FUNCTION "Gest Consensi" : VOID
TITLE =GESTIONE CONSENSI
AUTHOR : MassimoZ
VERSION : 0.1

BEGIN
NETWORK
TITLE ======== Consensi Prima Zona =======

NETWORK
TITLE =Cons Salita Testa Corto Circuito 1
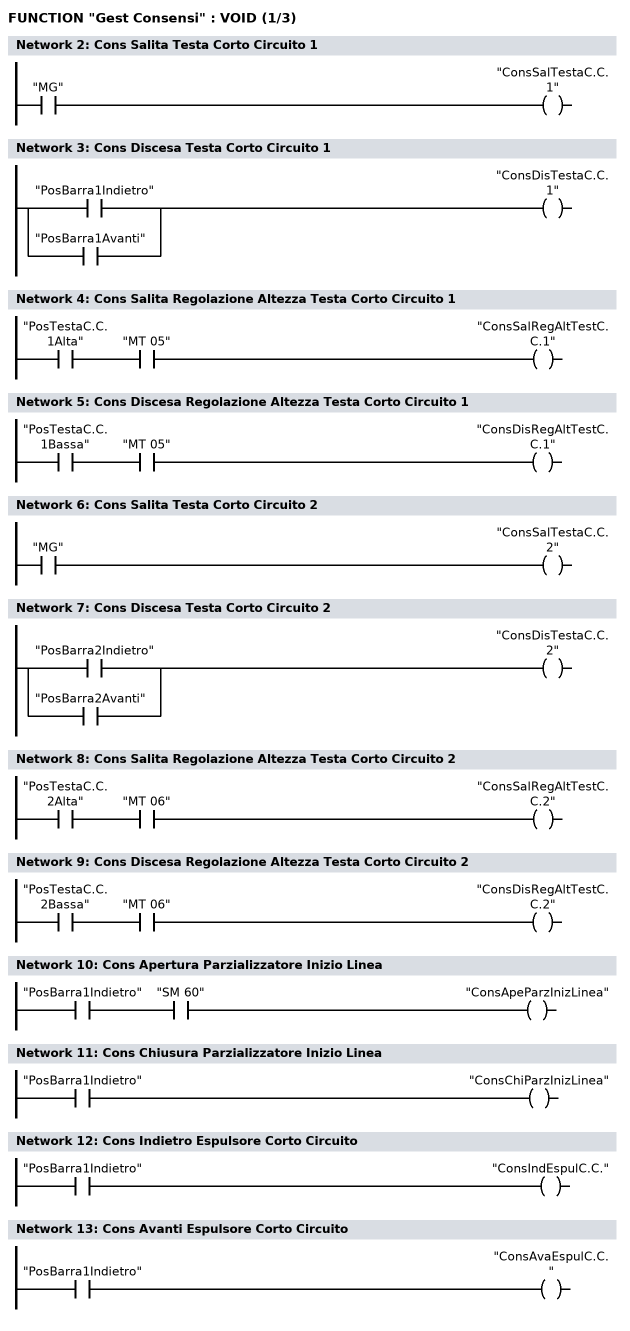
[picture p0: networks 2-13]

      U     "MG";
      =     "ConsSalTestaC.C.1";
NETWORK
TITLE =Cons Discesa Testa Corto Circuito 1

      O     "PosBarra1Indietro";
      O     "PosBarra1Avanti";
      =     "ConsDisTestaC.C.1";
NETWORK
TITLE =Cons Salita Regolazione Altezza Testa Corto Circuito 1

      U     "PosTestaC.C.1Alta";
      U     "MT 05";
      =     "ConsSalRegAltTestC.C.1";
NETWORK
TITLE =Cons Discesa Regolazione Altezza Testa Corto Circuito 1

      U     "PosTestaC.C.1Bassa";
      U     "MT 05";
      =     "ConsDisRegAltTestC.C.1";
NETWORK
TITLE =Cons Salita Testa Corto Circuito 2

      U     "MG";
      =     "ConsSalTestaC.C.2";
NETWORK
TITLE =Cons Discesa Testa Corto Circuito 2

      O     "PosBarra2Indietro";
      O     "PosBarra2Avanti";
      =     "ConsDisTestaC.C.2";
NETWORK
TITLE =Cons Salita Regolazione Altezza Testa Corto Circuito 2

      U     "PosTestaC.C.2Alta";
      U     "MT 06";
      =     "ConsSalRegAltTestC.C.2";
NETWORK
TITLE =Cons Discesa Regolazione Altezza Testa Corto Circuito 2

      U     "PosTestaC.C.2Bassa";
      U     "MT 06";
      =     "ConsDisRegAltTestC.C.2";
NETWORK
TITLE =Cons Apertura Parzializzatore Inizio Linea

      U     "PosBarra1Indietro";
      U     "SM 60";
      =     "ConsApeParzInizLinea";
NETWORK
TITLE =Cons Chiusura Parzializzatore Inizio Linea

      U     "PosBarra1Indietro";
      =     "ConsChiParzInizLinea";
NETWORK
TITLE =Cons Indietro Espulsore Corto Circuito

      U     "PosBarra1Indietro";
      =     "ConsIndEspulC.C.";
NETWORK
TITLE =Cons Avanti Espulsore Corto Circuito

      U     "PosBarra1Indietro";
      =     "ConsAvaEspulC.C.";
NETWORK
TITLE =Cons Indietro Barra 1
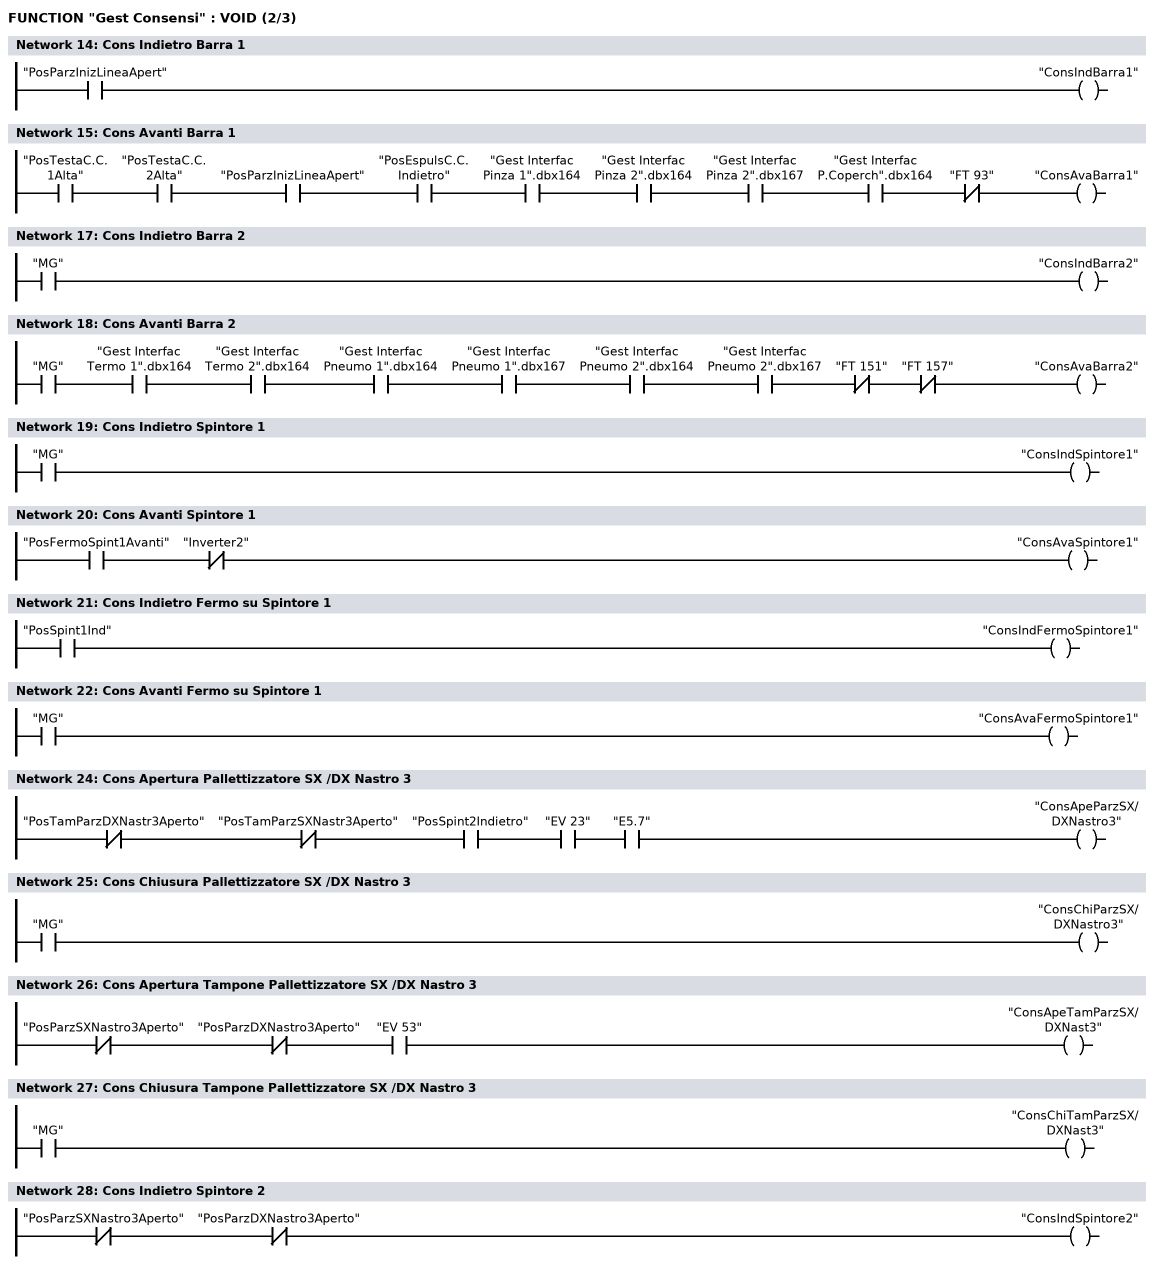
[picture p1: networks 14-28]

      U     "PosParzInizLineaApert";
      =     "ConsIndBarra1";
NETWORK
TITLE =Cons Avanti Barra 1

      U     "PosTestaC.C.1Alta";
      U     "PosTestaC.C.2Alta";
      U     "PosParzInizLineaApert";
      U     "PosEspulsC.C.Indietro";
      U     "Gest Interfac Pinza 1".dbx164;
      U     "Gest Interfac Pinza 2".dbx164;
      U     "Gest Interfac Pinza 2".dbx167;
      U     "Gest Interfac P.Coperch".dbx164;
      UN    "FT 93";
      =     "ConsAvaBarra1";
NETWORK
TITLE ======== Consensi Pulsantiera 1 =======

NETWORK
TITLE =Cons Indietro Barra 2

      U     "MG";
      =     "ConsIndBarra2";
NETWORK
TITLE =Cons Avanti Barra 2

      U     "MG";
      U     "Gest Interfac Termo 1".dbx164;
      U     "Gest Interfac Termo 2".dbx164;
      U     "Gest Interfac Pneumo 1".dbx164;
      U     "Gest Interfac Pneumo 1".dbx167;
      U     "Gest Interfac Pneumo 2".dbx164;
      U     "Gest Interfac Pneumo 2".dbx167;
      UN    "FT 151";
      UN    "FT 157";
      =     "ConsAvaBarra2";
NETWORK
TITLE =Cons Indietro Spintore 1

      U     "MG";
      =     "ConsIndSpintore1";
NETWORK
TITLE =Cons Avanti Spintore 1

      U     "PosFermoSpint1Avanti";
      UN    "Inverter2";
      =     "ConsAvaSpintore1";
NETWORK
TITLE =Cons Indietro Fermo su Spintore 1

      U     "PosSpint1Ind";
      =     "ConsIndFermoSpintore1";
NETWORK
TITLE =Cons Avanti Fermo su Spintore 1

      U     "MG";
      =     "ConsAvaFermoSpintore1";
NETWORK
TITLE ======== Consensi Pulsantiera 2 =======

NETWORK
TITLE =Cons Apertura Pallettizzatore SX /DX Nastro 3

      UN    "PosTamParzDXNastr3Aperto";
      UN    "PosTamParzSXNastr3Aperto";
      U     "PosSpint2Indietro";
      U     "EV 23";
      U     "E5.7";
      =     "ConsApeParzSX/DXNastro3";
NETWORK
TITLE =Cons Chiusura Pallettizzatore SX /DX Nastro 3

      U     "MG";
      =     "ConsChiParzSX/DXNastro3";
NETWORK
TITLE =Cons Apertura Tampone Pallettizzatore SX /DX Nastro 3

      UN    "PosParzSXNastro3Aperto";
      UN    "PosParzDXNastro3Aperto";
      U     "EV 53";
      =     "ConsApeTamParzSX/DXNast3";
NETWORK
TITLE =Cons Chiusura Tampone Pallettizzatore SX /DX Nastro 3

      U     "MG";
      =     "ConsChiTamParzSX/DXNast3";
NETWORK
TITLE =Cons Indietro Spintore 2

      UN    "PosParzSXNastro3Aperto";
      UN    "PosParzDXNastro3Aperto";
      =     "ConsIndSpintore2";
NETWORK
TITLE =Cons Avanti Spintore 2
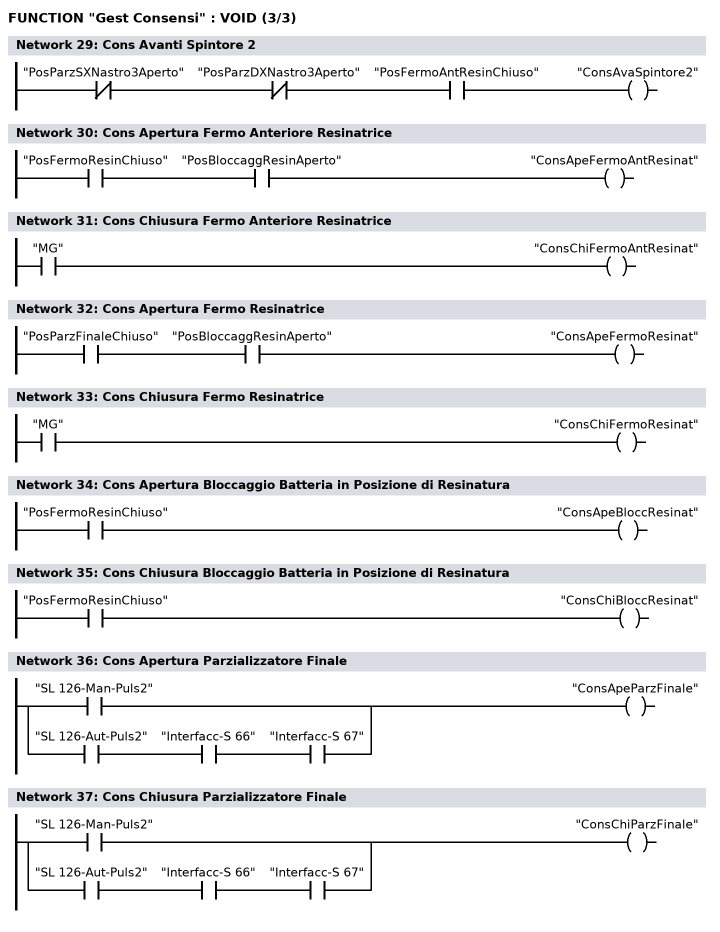
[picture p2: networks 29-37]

      UN    "PosParzSXNastro3Aperto";
      UN    "PosParzDXNastro3Aperto";
      U     "PosFermoAntResinChiuso";
      =     "ConsAvaSpintore2";
NETWORK
TITLE =Cons Apertura Fermo Anteriore Resinatrice

      U     "PosFermoResinChiuso";
      U     "PosBloccaggResinAperto";
      =     "ConsApeFermoAntResinat";
NETWORK
TITLE =Cons Chiusura Fermo Anteriore Resinatrice

      U     "MG";
      =     "ConsChiFermoAntResinat";
NETWORK
TITLE =Cons Apertura Fermo Resinatrice

      U     "PosParzFinaleChiuso";
      U     "PosBloccaggResinAperto";
      =     "ConsApeFermoResinat";
NETWORK
TITLE =Cons Chiusura Fermo Resinatrice

      U     "MG";
      =     "ConsChiFermoResinat";
NETWORK
TITLE =Cons Apertura Bloccaggio Batteria in Posizione di Resinatura

      U     "PosFermoResinChiuso";
      =     "ConsApeBloccResinat";
NETWORK
TITLE =Cons Chiusura Bloccaggio Batteria in Posizione di Resinatura

      U     "PosFermoResinChiuso";
      =     "ConsChiBloccResinat";
NETWORK
TITLE =Cons Apertura Parzializzatore Finale

      O     "SL 126-Man-Puls2";
      O     ;
      U     "SL 126-Aut-Puls2";
      U     "Interfacc-S 66";
      U     "Interfacc-S 67";
      =     "ConsApeParzFinale";
NETWORK
TITLE =Cons Chiusura Parzializzatore Finale

      O     "SL 126-Man-Puls2";
      O     ;
      U     "SL 126-Aut-Puls2";
      U     "Interfacc-S 66";
      U     "Interfacc-S 67";
      =     "ConsChiParzFinale";
END_FUNCTION

